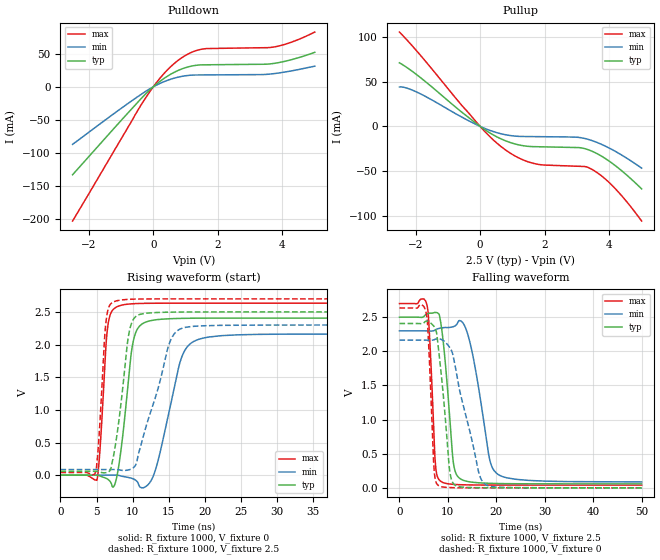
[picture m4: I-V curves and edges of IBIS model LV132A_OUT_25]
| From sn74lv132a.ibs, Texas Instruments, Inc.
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[Model]   LV132A_OUT_25
Model_type  Output
Vref =   0
Rref =   1000
Cref =   50p
Vmeas =   1.25
| variable   typ   min   max
C_comp   6.84pF   3.55pF   15.70pF
| C_pullup   5.33pF   3.55pF   7.61pF
| C_pulldown   8.35pF   4.05pF   15.70pF
[Temperature Range]   40   100   -40
| Ambient temperature   25   85   -40
[Voltage range]   2.5   2.3   2.7
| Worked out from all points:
|   slope of the pulldown table from 0 to 0.375 V, typ, clamps not added: 26.7 ohm
|   slope of the pullup table from 0 to 0.375 V, typ, clamps not added: 42 ohm
|   rising waveform, R_fixture 1000, V_fixture 0: 20-80 % time 1.39ns typ, 2.59ns min, 835ps max; typ from 0 V to 2.41 V
|   falling waveform, R_fixture 1000, V_fixture 2.5: 20-80 % time 1.66ns typ, 2.95ns min, 990ps max; typ from 2.5 V to 0.058 V
|   rising waveform, R_fixture 1000, V_fixture 2.5: 20-80 % time 1.54ns typ, 3.37ns min, 825ps max; typ from 0.058 V to 2.5 V
|   falling waveform, R_fixture 1000, V_fixture 0: 20-80 % time 1.84ns typ, 4.12ns min, 944ps max; typ from 2.41 V to 0 V
[Pulldown]
| LV132A_OUT_25
|   Voltage   I(typ)   I(min)   I(max)
-2.5V     -132.8mA   -86.91mA   -202.6mA
-1.085V   -55.61mA   -35.71mA   -86.07mA
-260mV    -11.9mA    -7.59mA    -18.35mA
10mV      425.4uA    265.2uA    665.9uA
250mV     9.806mA    6.028mA    15.48mA
500mV     17.9mA     10.82mA    28.56mA
745mV     24.18mA    14.32mA    39.05mA
1.105V    30.42mA    17.3mA     50.26mA
1.465V    33.09mA    17.9mA     56.46mA
3.71V     35.18mA    19.77mA    59.97mA
4.29V     41.16mA    24.16mA    67.63mA
5V        52.09mA    31.17mA    82.74mA
[Pullup]
| LV132A_OUT_25
|   Voltage   I(typ)   I(min)   I(max)
-2.5V     71.24mA    44.16mA    105.7mA
-2.26V    65.75mA    42.81mA    96.58mA
-1.89V    55.84mA    37.21mA    81.42mA
30mV      -796.3uA   -498.9uA   -1.231mA
665mV     -14.29mA   -8.401mA   -23.11mA
1.16V     -20.42mA   -11.08mA   -34.69mA
1.655V    -22.69mA   -11.42mA   -41.46mA
3.06V     -23.78mA   -12.37mA   -44.71mA
3.435V    -27.37mA   -15.55mA   -47.68mA
3.77V     -33.61mA   -20.32mA   -55.79mA
4.135V    -42.62mA   -26.97mA   -67.95mA
5V        -70.03mA   -46.75mA   -106mA
[Ramp]
| LV132A_OUT_25
| variable   typ   min   max
dV/dt_r   1.55/1.51E-09   1.41/2.83E-09   1.63/8.64E-10
dV/dt_f   1.51/1.72E-09   1.42/3.23E-09   1.64/1.02E-09
R_load = 1000
[Rising Waveform]
| LV132A_OUT_25
R_fixture =   1000
C_fixture =   0
L_fixture =   0
V_fixture =   0
V_fixture_min = 0
V_fixture_max = 0
|   Time   V(typ)   V(min)   V(max)
0s        1.615nV    9.162nV    1.013nV
5.055ns   113.2uV    -15.7uV    -75.99mV
6.51ns    -58.4mV    901.2uV    2.232V
7.865ns   1.687mV    -728uV     2.58V
9.985ns   1.987V     -51.75mV   2.625V
11.54ns   2.33V      -192.3mV   2.631V
13.3ns    2.38V      127.1mV    2.633V
16.73ns   2.401V     1.781V     2.634V
18.48ns   2.404V     2.048V     2.634V
50ns      2.406V     2.161V     2.634V
[Falling Waveform]
| LV132A_OUT_25
R_fixture =   1000
C_fixture =   0
L_fixture =   0
V_fixture =   2.5
V_fixture_min = 2.3
V_fixture_max = 2.7
|   Time   V(typ)   V(min)   V(max)
0s        2.5V       2.3V       2.7V
5.685ns   2.549V     2.299V     2.678V
7.4ns     2.569V     2.313V     373.7mV
8.505ns   2.433V     2.341V     97.14mV
11.07ns   402.9mV    2.361V     51.47mV
12.38ns   142mV      2.451V     46.43mV
14.59ns   87.13mV    2.121V     42.73mV
18.52ns   66.8mV     449.7mV    40.81mV
20ns      63.96mV    215.8mV    40.59mV
50ns      58.34mV    86.46mV    40.31mV
[Rising Waveform]
| LV132A_OUT_25
R_fixture =   1000
C_fixture =   0
L_fixture =   0
V_fixture =   2.5
V_fixture_min = 2.3
V_fixture_max = 2.7
|   Time   V(typ)   V(min)   V(max)
0s        58.33mV    86.01mV    40.31mV
4.885ns   59.52mV    86.03mV    49.69mV
5.32ns    53.36mV    86.01mV    539.7mV
6.28ns    37.91mV    86.62mV    2.312V
7.31ns    265.7mV    86.93mV    2.651V
9.445ns   2.139V     80.71mV    2.692V
10.74ns   2.45V      286.3mV    2.697V
15.02ns   2.496V     1.991V     2.7V
16.63ns   2.498V     2.24V      2.7V
50ns      2.5V       2.3V       2.7V
[Falling Waveform]
| LV132A_OUT_25
R_fixture =   1000
C_fixture =   0
L_fixture =   0
V_fixture =   0
V_fixture_min = 0
V_fixture_max = 0
|   Time   V(typ)   V(min)   V(max)
0s        2.408V     2.164V     2.635V
5.505ns   2.442V     2.164V     2.565V
5.97ns    2.439V     2.163V     2.188V
7.14ns    2.365V     2.169V     289.3mV
7.995ns   2.083V     2.186V     37mV
10.32ns   281.9mV    2.063V     4.666mV
11.44ns   41.46mV    1.807V     2.549mV
16.32ns   2.72mV     239mV      319.8uV
17.75ns   1.8mV      49.75mV    182uV
50ns      501.3nV    46.21uV    169.7nV
